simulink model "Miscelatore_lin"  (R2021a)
settings: Solver=VariableStepAuto  StartTime=0.0  StopTime=10000  MaxStep=1  RelTol=1e-3
undefined symbols (not defined in the file or in its folder): A, Avds, Bvds, cv, cvm, Evds, h, Mm, P, rho, Rma, T0, T1star, T2star, Tamb, Tm0, Tmstar, Tstar, w1star, w2star, wstar, z0, zstar

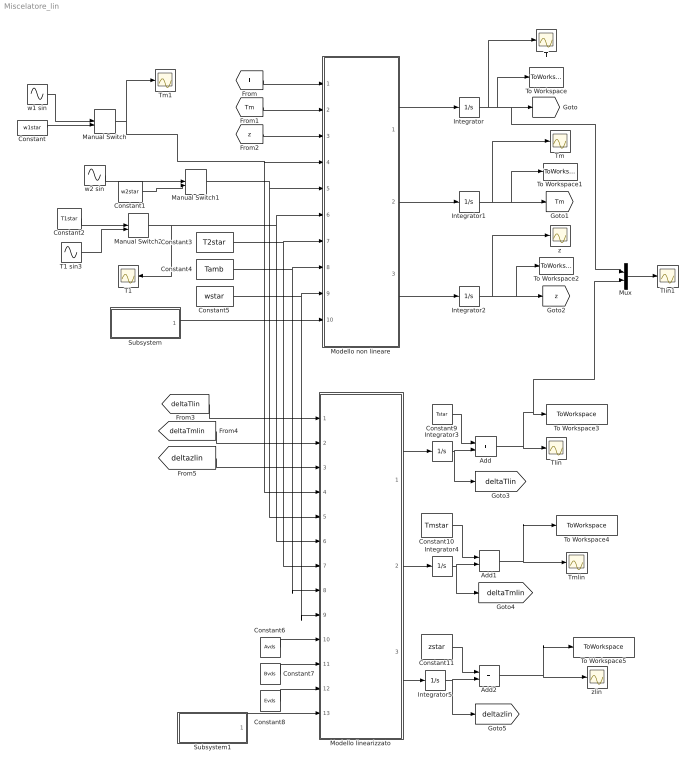
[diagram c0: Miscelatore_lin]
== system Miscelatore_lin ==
  Add : Sum
  Add1 : Sum
  Add2 : Sum
  Constant : Constant  Value=w1star
  Constant1 : Constant  Value=w2star
  Constant10 : Constant  Value=Tmstar
  Constant11 : Constant  Value=zstar
  Constant2 : Constant  Value=T1star
  Constant3 : Constant  Value=T2star
  Constant4 : Constant  Value=Tamb
  Constant5 : Constant  Value=wstar
  Constant6 : Constant  Value=Avds
  Constant7 : Constant  Value=Bvds
  Constant8 : Constant  Value=Evds
  Constant9 : Constant  Value=Tstar
  Integrator : Integrator  InitialCondition=T0
  Integrator1 : Integrator  InitialCondition=Tm0
  Integrator2 : Integrator  InitialCondition=z0
  Integrator3 : Integrator  InitialCondition=T0-Tstar
  Integrator4 : Integrator  InitialCondition=Tm0-Tmstar
  Integrator5 : Integrator  InitialCondition=z0-zstar
  Manual Switch : ManualSwitch
  Manual Switch1 : ManualSwitch
  Manual Switch2 : ManualSwitch  CurrentSetting=0
  Modello linearizzato : MATLAB Function  TreatAsAtomicUnit=on
  Modello non lineare : MATLAB Function  TreatAsAtomicUnit=on
  Mux : Mux  Inputs=2
  Subsystem : Subsystem
  Subsystem1 : Subsystem
  T : Scope
  T1 : Scope
  T1 sin3 : Sin  Amplitude=T1star/2  Bias=T1star  Frequency=0.001  SampleTime=0
  Tlin : Scope
  Tlin1 : Scope
  Tm : Scope
  Tm1 : Scope
  Tmlin : Scope
  To Workspace : ToWorkspace  VariableName=T  SaveFormat=Timeseries  SampleTime=-1
  To Workspace1 : ToWorkspace  VariableName=Tm  SaveFormat=Timeseries  SampleTime=-1
  To Workspace2 : ToWorkspace  VariableName=z  SaveFormat=Timeseries  SampleTime=-1
  To Workspace3 : ToWorkspace  VariableName=Tlin  SaveFormat=Timeseries  SampleTime=-1
  To Workspace4 : ToWorkspace  VariableName=Tmlin  SaveFormat=Timeseries  SampleTime=-1
  To Workspace5 : ToWorkspace  VariableName=zlin  SaveFormat=Timeseries  SampleTime=-1
  w1 sin : Sin  Amplitude=0.6*w1star  Bias=w1star  Frequency=0.001  SampleTime=0
  w2 sin : Sin  Amplitude=0.1*w2star  Bias=w2star  Frequency=0.002  SampleTime=0
  z : Scope
  zlin : Scope
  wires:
  Modello non lineare/1(Tdot) -> Integrator/1
  Modello non lineare/2(Tmdot) -> Integrator1/1
  Modello non lineare/3(zdot) -> Integrator2/1
  Integrator/1 -> T/1, To Workspace/1, Mux/1, [T]
  Integrator1/1 -> Tm/1, To Workspace1/1, [Tm]
  Integrator2/1 -> z/1, To Workspace2/1, [z]
  [T] -> Modello non lineare/1(T)
  [Tm] -> Modello non lineare/2(Tm)
  [z] -> Modello non lineare/3(z)
  Subsystem/1(par) -> Modello non lineare/10(par)
  Manual Switch/1 -> Modello non lineare/4(w1), Modello linearizzato/4(w1), Tm1/1
  Manual Switch1/1 -> Modello linearizzato/5(w2), Modello non lineare/5(w2)
  Manual Switch2/1 -> T1/1, Modello linearizzato/6(T1), Modello non lineare/6(T1)
  Constant3/1 -> Modello non lineare/7(T2), Modello linearizzato/7(T2)
  Constant4/1 -> Modello linearizzato/8(Tamb), Modello non lineare/8(Tamb)
  Constant5/1 -> Modello linearizzato/9(w), Modello non lineare/9(w)
  Modello linearizzato/1(deltaTdot) -> Integrator3/1
  Modello linearizzato/2(deltaTmdot) -> Integrator4/1
  Modello linearizzato/3(deltazdot) -> Integrator5/1
  Constant6/1 -> Modello linearizzato/10(Avds)
  Constant7/1 -> Modello linearizzato/11(Bvds)
  Constant8/1 -> Modello linearizzato/12(Evds)
  [deltaTlin] -> Modello linearizzato/1(deltaT)
  [deltaTmlin] -> Modello linearizzato/2(deltaTm)
  [deltazlin] -> Modello linearizzato/3(deltaz)
  Subsystem1/1(par) -> Modello linearizzato/13(par)
  Integrator3/1 -> [deltaTlin], Add/2
  Constant9/1 -> Add/1
  Integrator4/1 -> [deltaTmlin], Add1/2
  Constant10/1 -> Add1/1
  Integrator5/1 -> [deltazlin], Add2/2
  Constant11/1 -> Add2/1
  Add/1 -> Mux/2, To Workspace3/1, Tlin/1
  Add1/1 -> To Workspace4/1, Tmlin/1
  Add2/1 -> To Workspace5/1, zlin/1
  Mux/1 -> Tlin1/1
  w1 sin/1 -> Manual Switch/1
  Constant/1 -> Manual Switch/2
  Constant1/1 -> Manual Switch1/2
  w2 sin/1 -> Manual Switch1/1
  Constant2/1 -> Manual Switch2/1
  T1 sin3/1 -> Manual Switch2/2

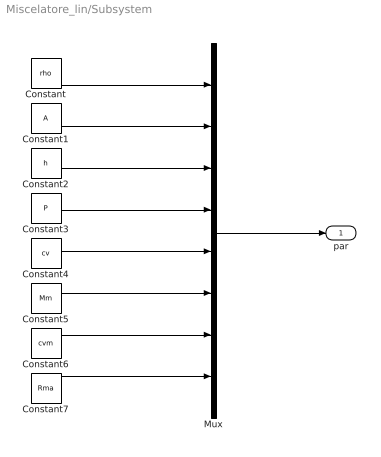
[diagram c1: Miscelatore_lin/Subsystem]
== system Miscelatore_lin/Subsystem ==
  Constant : Constant  Value=rho
  Constant1 : Constant  Value=A
  Constant2 : Constant  Value=h
  Constant3 : Constant  Value=P
  Constant4 : Constant  Value=cv
  Constant5 : Constant  Value=Mm
  Constant6 : Constant  Value=cvm
  Constant7 : Constant  Value=Rma
  Mux : Mux  Inputs=8
  par : Outport
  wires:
  Constant/1 -> Mux/1
  Constant1/1 -> Mux/2
  Constant2/1 -> Mux/3
  Constant3/1 -> Mux/4
  Constant4/1 -> Mux/5
  Constant5/1 -> Mux/6
  Constant6/1 -> Mux/7
  Constant7/1 -> Mux/8
  Mux/1 -> par/1

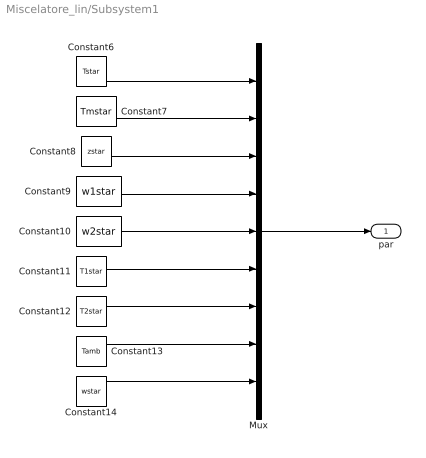
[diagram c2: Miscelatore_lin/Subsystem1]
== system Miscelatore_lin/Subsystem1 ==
  Constant10 : Constant  Value=w2star
  Constant11 : Constant  Value=T1star
  Constant12 : Constant  Value=T2star
  Constant13 : Constant  Value=Tamb
  Constant14 : Constant  Value=wstar
  Constant6 : Constant  Value=Tstar
  Constant7 : Constant  Value=Tmstar
  Constant8 : Constant  Value=zstar
  Constant9 : Constant  Value=w1star
  Mux : Mux  Inputs=9
  par : Outport
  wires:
  Constant12/1 -> Mux/7
  Mux/1 -> par/1
  Constant6/1 -> Mux/1
  Constant9/1 -> Mux/4
  Constant11/1 -> Mux/6
  Constant13/1 -> Mux/8
  Constant8/1 -> Mux/3
  Constant10/1 -> Mux/5
  Constant7/1 -> Mux/2
  Constant14/1 -> Mux/9

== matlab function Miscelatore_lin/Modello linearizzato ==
function [deltaTdot,deltaTmdot,deltazdot] = fcn(deltaT,deltaTm,deltaz,w1,w2,T1,T2,Tamb,w,Avds,Bvds,Evds,par)

Tstar=par(1);
Tmstar=par(2);
zstar=par(3);
w1star=par(4);
w2star=par(5);
T1star=par(6);
T2star=par(7);
Tambstar=par(8);
wstar=par(9);

deltaX=[deltaT;deltaTm;deltaz];
deltaU=[w1-w1star;w2-w2star];
deltaD=[T1-T1star;T2-T2star;Tamb-Tambstar;w-wstar];

deltaXdot=Avds*deltaX+Bvds*deltaU+Evds*deltaD;

deltaTdot=deltaXdot(1);
deltaTmdot=deltaXdot(2);
deltazdot=deltaXdot(3);

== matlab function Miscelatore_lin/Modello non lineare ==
function [Tdot,Tmdot,zdot] = fcn(T,Tm,z,w1,w2,T1,T2,Tamb,w,par)

rho=par(1);
A=par(2);
h=par(3);
P=par(4);
cv=par(5);
Mm=par(6);
cvm=par(7);
Rma=par(8);

%Tdot=-((w1+w2)/(rho*A*z)+h*P/(rho*cv*A))*T+h*P/(rho*cv*A)*Tm+w1*T1/(rho*A*z)+w2*T2/(rho*A*z);

Tdot=w1/(rho*A*z)*(T1-T)+w2/(rho*A*z)*(T2-T)-h*P/(rho*cv*A)*(T-Tm);

Tmdot=-(h*P*z/(Mm*cvm)+1/(Mm*cvm*Rma))*Tm+h*P*z/(Mm*cvm)*T+Tamb/(Mm*cvm*Rma);

zdot=(w1+w2-w)/(rho*A);
